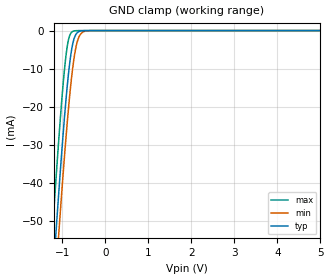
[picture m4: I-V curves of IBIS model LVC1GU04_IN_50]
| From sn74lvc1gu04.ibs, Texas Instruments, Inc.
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[Model]   LVC1GU04_IN_50
Model_type  Input
Vinl=1.125
Vinh=4.125
| variable   typ   min   max
C_comp   4.33pF   2.71pF   5.09pF
[Temperature Range]   40   100   -40
| Ambient temperature   25   85   -40
[Voltage range]   5   4.5   5.5
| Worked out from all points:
|   GND clamp passes 1 mA (typ) near -0.68 V on its own axis
[GND Clamp]
| LVC1GU04_IN_50
|   Voltage   I(typ)   I(min)   I(max)
-5.5V     -872.3mA   -880mA     -863mA
-1.25V    -71.03mA   -81.88mA   -57.11mA
-1.22V    -65.92mA   -76.78mA   -51.96mA
-1.14V    -52.55mA   -63.42mA   -38.55mA
-1.075V   -42.06mA   -52.87mA   -28.16mA
-980mV    -27.63mA   -38.14mA   -14.46mA
-905mV    -17.45mA   -27.36mA   -6.068mA
-835mV    -9.584mA   -18.33mA   -1.666mA
-750mV    -3.29mA    -9.411mA   -201uA
-625mV    -352.4uA   -2.117mA   -6.8uA
-455mV    -11.52uA   -138.5uA   -65.59nA
5V        1.117nA    59.61nA    9.482pA
